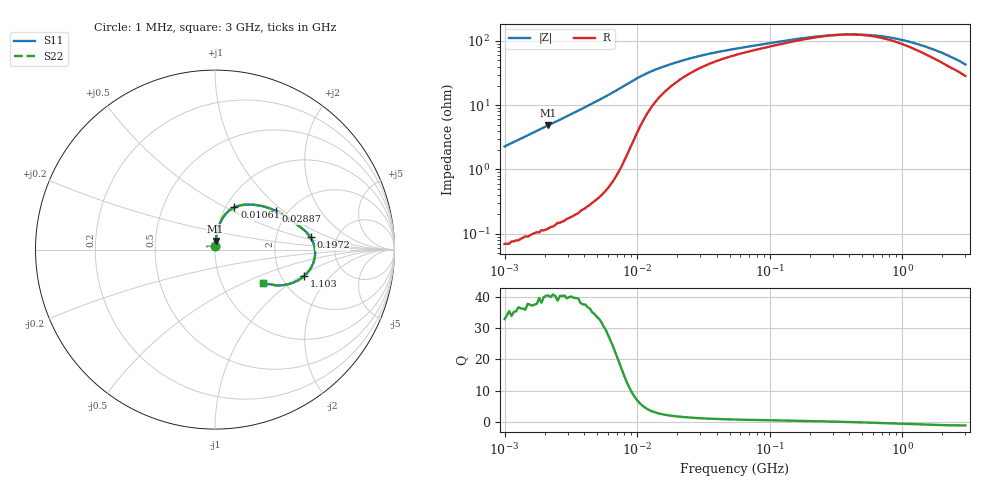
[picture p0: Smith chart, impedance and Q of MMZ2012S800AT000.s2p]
! S-parameter Generated by TDK Corporation
! Copyright(C) 2016 TDK Corporation.
! All Rights Reserved.
! TDK P/N: MMZ2012S800AT000 (Chip Beads)
! Property: |Z|=80¶ at 100MHz
! Size(LxWxT): 2x1.25x0.85mm, 0.079x0.049x0.033inches
! Model Type: s2p (Touchstone File Format Version 1.0)
! Frequency: DC=Yes Start=1MHz Stop=3000MHz 202points Log-sweep
! Note: This model was converted from impedance.
! Model Generated on May. 16, 2016
! Hash(MD5):
! Port Assignments:
!  1 ---@@@--- 2
! Applicable Conditions:
!  Temperature = 25 degC
!  DC Bias Current = 0 A
!  Small Signal Operation
! Terms and conditions regarding TDK Simulation Models
! (1)This simulation model is being provided solely for informational purposes. Please refer to the specifications of the products in terms of detailed characteristics of such products.
! (2)In no event shall TDK Corporation of any of its subsidiaries be liable for any loss or damage arising, directly or indirectly,
!  From any information contained in this simulation model, including, but not limited to loss or damages arising from any inaccuracies, omissions or errors in connection with such information.
! (3)Any and all copyrights on this simulation model are owned by TDK Corporation.
!  Duplication or redistribution of this simulation model without prior written permission from TDK Corporation is prohibited.
! (4)This simulation model is subject to any modification or change without any prior notice.
! (5)Neither TDK Corporation nor any of its subsidiaries shall make any warranty, express or implied,
!  Including but not limited to the correctness, implied warranties of merchantability and fitness for a particular purpose with respect to this simulation models.
! (6)The use of this simulation model shall be deemed to have consented to the terms and conditions hereof.
# MHz S MA R 50
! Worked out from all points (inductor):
!   201 points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, 1 MHz to 3 GHz, reference 50 ohm
!   read as one part in series: L = 362 nH near 1.041 MHz
!   highest Q = 40.3 at 2.14 MHz (marker M1), where L = 362 nH
!   self-resonance near 370 MHz
!   S11 on the Smith chart (normalised r, x): 1 MHz: 1.00, +0.05; 10.61 MHz: 1.10, +0.55; 28.87 MHz: 1.73, +0.89; 197.2 MHz: 3.19, +0.61; 1.103 GHz: 2.66, -1.07; 3 GHz: 1.57, -0.65
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1  0.02277 87.0  0.999 -1.3  0.999 -1.3  0.02277 87.0
2.13957  0.04853 85.8  0.9976 -2.8  0.9976 -2.8  0.04853 85.8
3.900413  0.08909 83.4  0.9937 -5.1  0.9937 -5.1  0.08909 83.4
5.372736  0.1246 81.0  0.9883 -7.2  0.9883 -7.2  0.1246 81.0
7.110411  0.1699 77.4  0.9771 -9.8  0.9771 -9.8  0.1699 77.4
8.686058  0.2128 72.7  0.9583 -12.2  0.9583 -12.2  0.2128 72.7
10.61086  0.2589 65.3  0.9225 -14.8  0.9225 -14.8  0.2589 65.3
14.61624  0.3174 52.3  0.8441 -17.3  0.8441 -17.3  0.3174 52.3
20.13356  0.3612 41.8  0.7694 -18.2  0.7694 -18.2  0.3612 41.8
28.86629  0.4014 32.5  0.6956 -18.0  0.6956 -18.0  0.4014 32.5
54.77226  0.4528 21.2  0.6007 -15.8  0.6007 -15.8  0.4528 21.2
197.1969  0.5365 7.3  0.4728 -8.3  0.4728 -8.3  0.5365 7.3
213.6344  0.5404 6.4  0.467 -7.5  0.467 -7.5  0.5404 6.4
318.8066  0.5543 1.8  0.4463 -2.3  0.4463 -2.3  0.5543 1.8
439.1493  0.5583 -2.2  0.4426 2.8  0.4426 2.8  0.5583 -2.2
581.181  0.5557 -6.1  0.4513 7.5  0.4513 7.5  0.5557 -6.1
800.5644  0.5433 -11.0  0.4782 12.6  0.4782 12.6  0.5433 -11.0
1102.76  0.5179 -16.6  0.5249 16.4  0.5249 16.4  0.5179 -16.6
1459.42  0.4824 -21.8  0.5802 17.9  0.5802 17.9  0.4824 -21.8
1931.433  0.4339 -27.0  0.6444 17.8  0.6444 17.8  0.4339 -27.0
2556.106  0.3691 -31.8  0.7133 15.8  0.7133 15.8  0.3691 -31.8
3000  0.3249 -34.4  0.7547 14.1  0.7547 14.1  0.3249 -34.4
